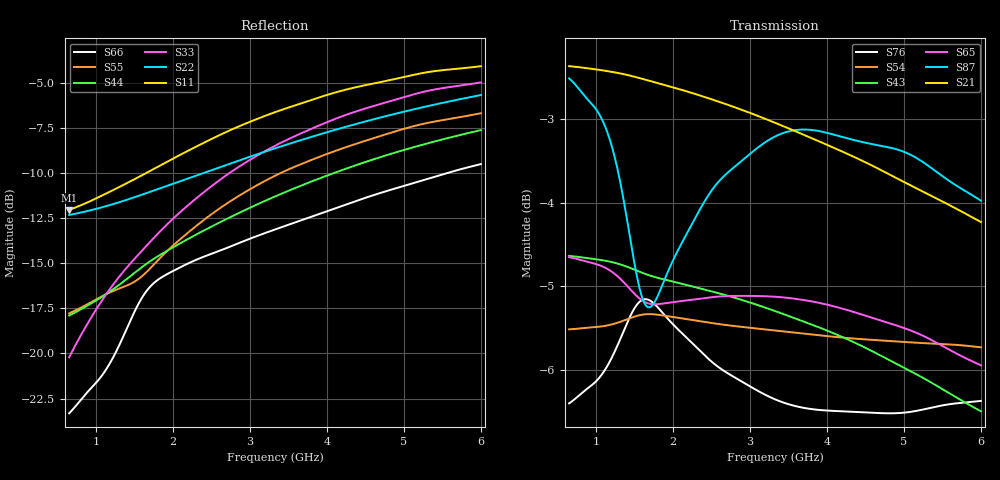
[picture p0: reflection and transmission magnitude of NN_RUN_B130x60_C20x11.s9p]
! IGNION VIRTUAL ANTENNA LIBRARY
! NN_RUN_B130x60_C20x11
! Virtual Antenna™ RUN mXTEND™: NN02-224 12.0 mm x 3.0 mm x 2.4 mm
! https://ignion.io/product/run-mxtend/
! Board: 130 mm x 60 mm
! Clearance Area: 20 mm x 11 mm
! Feeding line: L-shape; 11mm x 2mm and 5mm x 2mm
! Applications: Smartphone, Fleet management, IoT
! Frequency range 0.65GHz to 6GHz, step 10MHz
! Number of ports 9
! This product and its use is protected by at least one or more of the following patents and patent
! applications US 8,203,492 B2; US 8,237,615 B2; PCT/EP2013/064692; WO 2014/012842 A1; US 2019/190122 A1;
! US 62/072,671; and other domestic and international patents pending. Additional information about
! patents related to this product is available at https://ignion.io/files/Patent-list-NN.pdf, all
! rights reserved. Copyright, Ignion 2021.
! Need more help? Your platform is much different than these examples in the manual? Use our
! Fast Track service (https://ignion.io/fast-track/), for free, and get a personalized antenna design in
! just 24 hours.
! Touchstone port 1 = "Series Port"
! Touchstone port 2 = "Shunt Port"
! Touchstone port 3 = "Series Port"
! Touchstone port 4 = "Shunt Port"
! Touchstone port 5 = "Series Port"
! Touchstone port 6 = "Shunt Port"
! Touchstone port 7 = "Series Port"
! Touchstone port 8 = "Shunt Port"
! Touchstone port 9 = "Series Port"
! IE3D S-Parameters Output Version 2.0
# GHZ S MA R 50
! Nport = 9
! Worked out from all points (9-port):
!   536 points, 650 MHz to 6 GHz, reference 50 ohm
!   strongest paths, dB at 650 MHz, 1.99 GHz, 3.33 GHz, 4.67 GHz, 6 GHz:
!     S21: -2.4, -2.6, -3.0, -3.6, -4.2
!     S87: -2.5, -4.7, -3.2, -3.3, -4.0
!     S65: -4.7, -5.2, -5.1, -5.4, -5.9
!     S43: -4.6, -4.9, -5.3, -5.8, -6.5
!     S54: -5.5, -5.4, -5.5, -5.6, -5.7
!     S76: -6.4, -5.4, -6.4, -6.5, -6.4
!   lowest |S11| = -12.0 dB at 650 MHz (marker M1), VSWR 1.67, Z = 31.1 + j7.73 ohm
!   |S11| at or under -10 dB: start of sweep to 1.651 GHz
